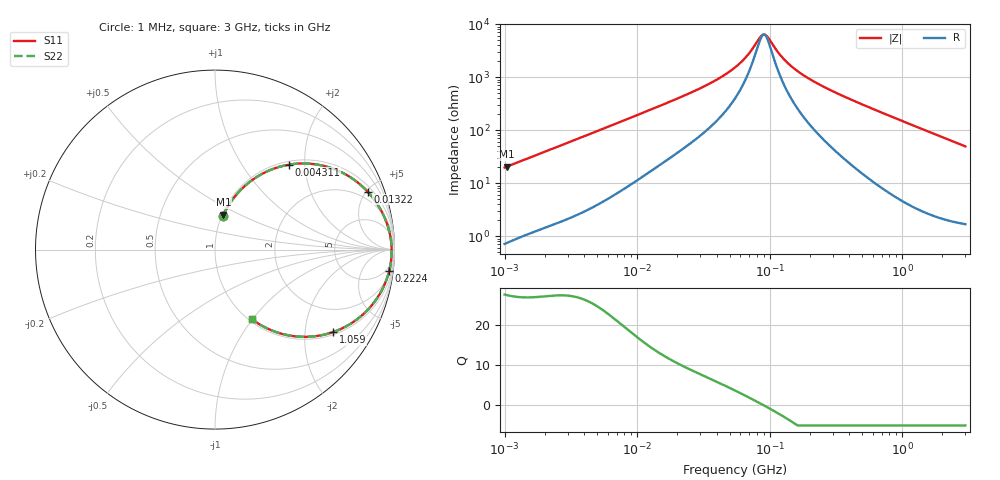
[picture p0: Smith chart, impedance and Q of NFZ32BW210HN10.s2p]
! NFZ32BW210HN10
# Hz S RI R 50
!Freq.(Hz) S11(Real) S11(Imag) S21(Real) S21(Imag) S12(Real) S12(Imag) S22(Real) S22(Imag)
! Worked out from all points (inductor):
!   401 points, 1 MHz to 3 GHz, reference 50 ohm
!   read as one part in series: L = 3.12 uH near 1.041 MHz
!   highest Q = 27.5 at 1.041 MHz (marker M1), where L = 3.14 uH
!   self-resonance near 90.51 MHz
!   S11 on the Smith chart (normalised r, x): 1 MHz: 1.01, +0.39; 4.311 MHz: 1.06, +1.66; 13.22 MHz: 1.36, +5.08; 222.4 MHz: 3, -16; 1.059 GHz: 1.08, -2.81; 3 GHz: 1.03, -0.99
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1000000  0.0439 0.1875  0.9561 -0.1875  0.9561 -0.1875  0.0439 0.1875
1040844  0.047 0.1943  0.953 -0.1943  0.953 -0.1943  0.047 0.1943
2097170  0.1512 0.3404  0.8488 -0.3404  0.8488 -0.3404  0.1512 0.3404
3823119  0.3567 0.4606  0.6433 -0.4606  0.6433 -0.4606  0.3567 0.4606
4310966  0.411 0.4731  0.589 -0.4731  0.589 -0.4731  0.411 0.4731
6969505  0.6356 0.4582  0.3644 -0.4582  0.3644 -0.4582  0.6356 0.4582
1.322427e7  0.8496 0.3236  0.1504 -0.3236  0.1504 -0.3236  0.8496 0.3236
1.461624e7  0.8707 0.2996  0.1293 -0.2996  0.1293 -0.2996  0.8707 0.2996
3.254976e7  0.9608 0.1367  0.0392 -0.1367  0.0392 -0.1367  0.9608 0.1367
5.477226e7  0.9794 0.0612  0.0206 -0.0612  0.0206 -0.0612  0.9794 0.0612
6.826239e7  0.9828 0.0336  0.0172 -0.0336  0.0172 -0.0336  0.9828 0.0336
8.507507e7  0.9844 0.00732  0.0156 -0.00732  0.0156 -0.00732  0.9844 0.00732
9.216659e7  0.9846 -0.00215  0.0154 0.00215  0.0154 0.00215  0.9846 -0.00215
9.787053e7  0.9846 -0.00926  0.0154 0.00926  0.0154 0.00926  0.9846 -0.00926
1.348146e8  0.9826 -0.0484  0.0174 0.0484  0.0174 0.0484  0.9826 -0.0484
2.094008e8  0.9726 -0.1103  0.0274 0.1103  0.0274 0.1103  0.9726 -0.1103
2.223601e8  0.9703 -0.1199  0.0297 0.1199  0.0297 0.1199  0.9703 -0.1199
4.570858e8  0.9068 -0.2651  0.0932 0.2651  0.0932 0.2651  0.9068 -0.2651
8.005644e8  0.7697 -0.404  0.2303 0.404  0.2303 0.404  0.7697 -0.404
1.059487e9  0.6592 -0.4591  0.3408 0.4591  0.3408 0.4591  0.6592 -0.4591
1.712864e9  0.43 -0.4812  0.57 0.4812  0.57 0.4812  0.43 -0.4812
3e9  0.2037 -0.386  0.7963 0.386  0.7963 0.386  0.2037 -0.386
